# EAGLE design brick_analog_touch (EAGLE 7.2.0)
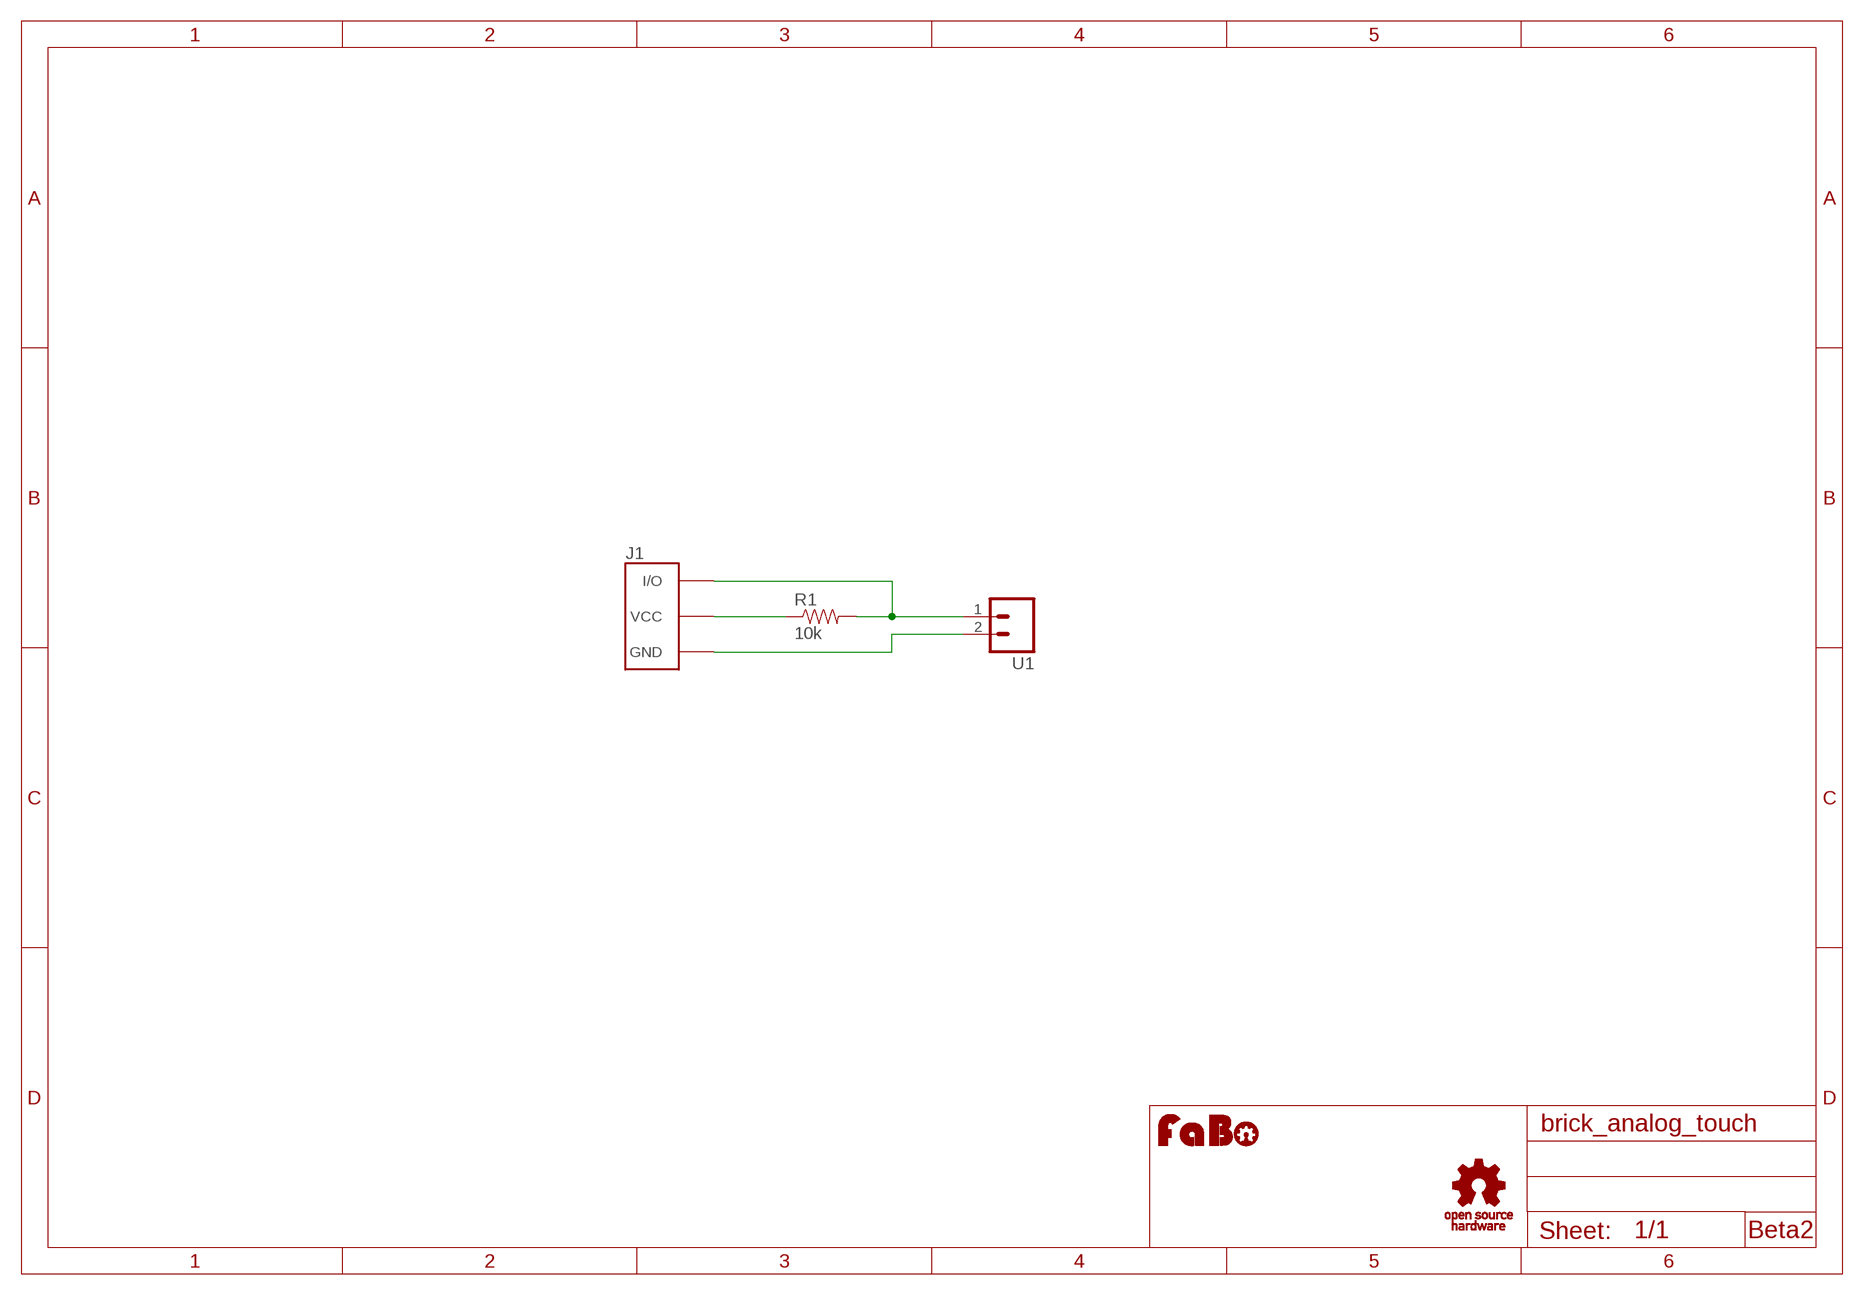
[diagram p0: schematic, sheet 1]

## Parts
J1  BRICK_3PIN  [BRICK_3PIN]
R1  10k  RES-PTH-REGULAR  [RES-AXL-REGULAR]
U1  M02LOCK  [1X02_LOCK]
U$2  LOGO_OSHW_T-M  [LOGO_OSHW_T_M]
U$3  LOGO_FABO-M  [LOGO_FABO_M]

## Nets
GND: J1.GND U1.2
N$1: J1.IN/OUT(I/O) R1.P$2 U1.1
N$2: J1.VCC R1.P$1

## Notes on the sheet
- Beta2

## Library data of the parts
J1 = Gclue:BRICK_3PIN: FaBo Brick 3pin
R1 = Gclue:RES
U1 = SparkFun:M02: Header 2
U$2 = Gclue:LOGO_OSHW_T
U$3 = FaBo:LOGO_FABO

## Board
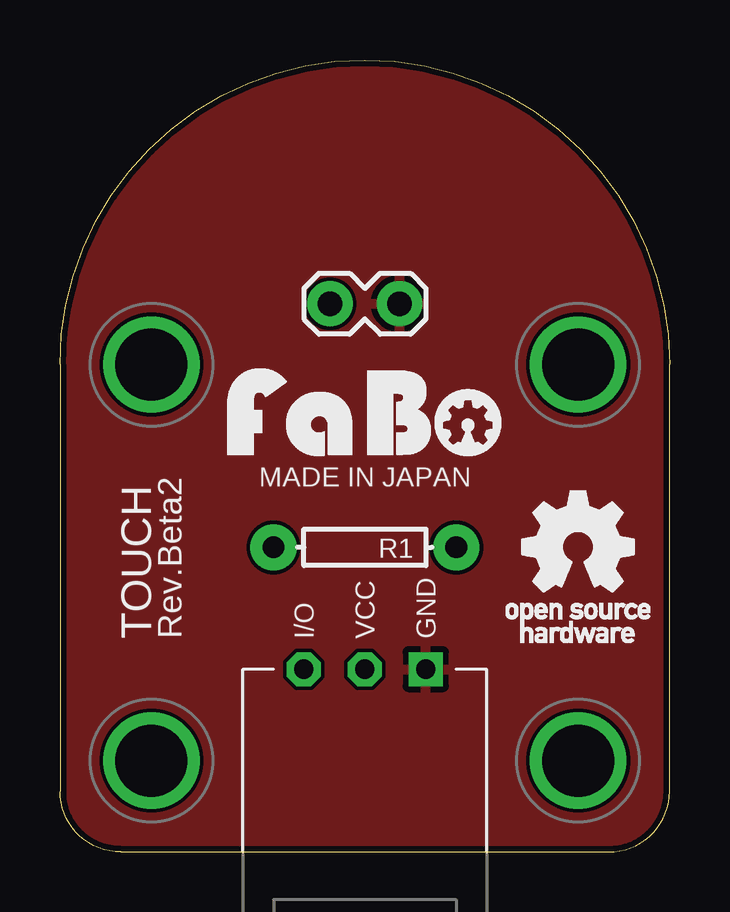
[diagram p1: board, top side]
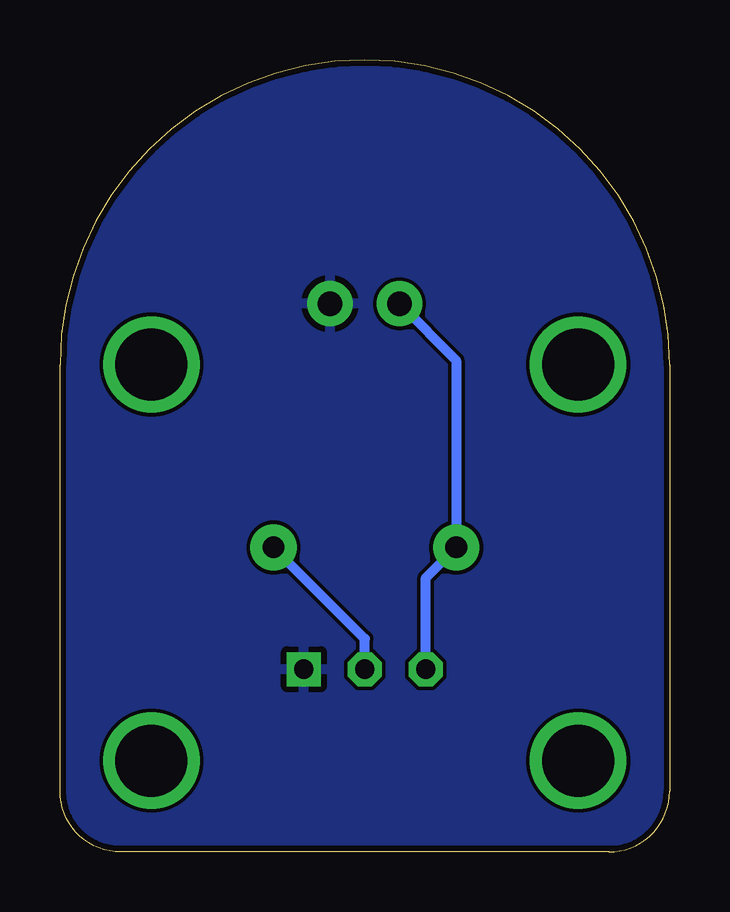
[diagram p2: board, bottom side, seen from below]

Size 25.4 x 33.02 mm. Coordinates in mm from the lower left corner, seen from the top.
Copper layers (1*16): Top 0.035mm / dielectric 1.5mm / Bottom 0.035mm
Design rules "Elecrow_2-layer_eagle_rule": minimum track width 6mil, minimum drill 12mil, track to track 6mil, track to pad 6mil, pad to pad 6mil, via to via 6mil, smd to smd 0mil, copper to edge 10mil, drill to drill 10mil, minimum pad ring 10mil, minimum via ring 6mil, stop-mask expansion 2mil, vias tented up to drill 100mil, thermal gap 10mil

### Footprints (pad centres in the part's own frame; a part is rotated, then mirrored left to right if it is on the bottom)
BRICK_3PIN = drill 0.8 pad 1.422 square: GND 2.54,-8.89 | drill 0.8 pad 1.422 octagon: IN/OUT -2.54,-8.89; VCC 0,-8.89 | drill 3 pad 3.81: P$5 -8.89,3.81; P$6 8.89,3.81; P$7 -8.89,-12.7; P$8 8.89,-12.7
RES-AXL-REGULAR = drill 0.9 pad 1.93: P$1 -3.81,0; P$2 3.81,0
1X02_LOCK = drill 1.016 pad 1.88: 1 -0.178,0; 2 2.718,0

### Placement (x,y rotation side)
J1  12.7,16.51 0 top
R1  12.7,12.7 180 top
U1  11.43,22.86 0 top
U$2  21.59,12.7 0 top
U$3  12.7,16.51 0 top

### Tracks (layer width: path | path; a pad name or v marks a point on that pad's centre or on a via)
GND
  pour Bottom: -1.27,-1.27 26.67,-1.27 26.67,34.29 -1.27,34.29
  pour Top: -1.27,-1.27 26.67,-1.27 26.67,34.29 -1.27,34.29
N$1
  Bottom 0.406: J1.IN/OUT 10.16,11.43 R1.P$2 8.89,20.5 U1.1
N$2
  Bottom 0.406: J1.VCC 12.7,8.89 R1.P$1

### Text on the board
tPlace: MADE IN JAPAN | TOUCH | Rev.Beta2

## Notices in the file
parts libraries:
SparkFun: Licensing: CC v3.0 Share-Alike You are welcome to use this library for commercial purposes.
